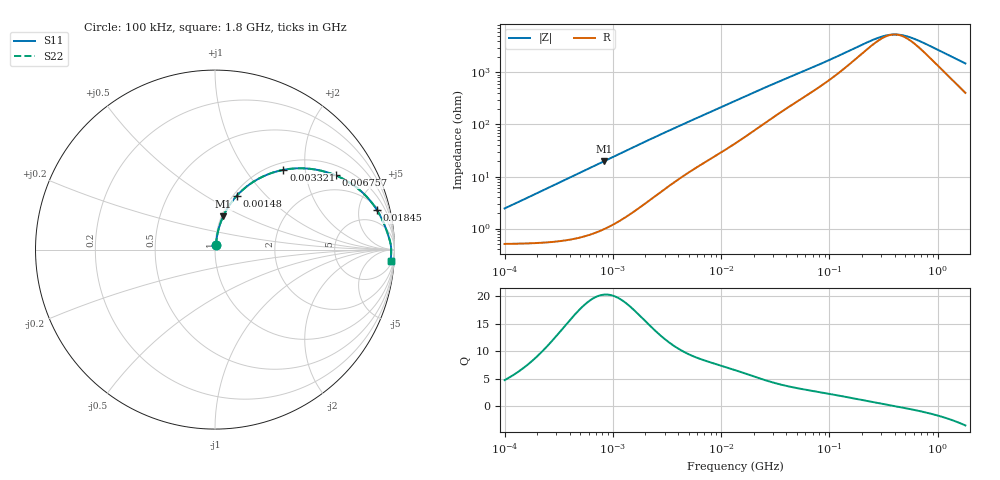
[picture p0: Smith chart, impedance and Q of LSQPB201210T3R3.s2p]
! LSQPB201210T3R3  S-PARAMETER MODEL  ( General Type )
! Model Generated by TAIYO YUDEN Corporation (http://www.ty-top.com)
! Version 2.0
! TAIYO YUDEN Control No. 100810NF18SB-HKC
! Copyright(c) 2007 TAIYO YUDEN CO.,LTD. All Rights Reserved.
! Product Description (link to TY-COMPAS)
! https://ds.yuden.co.jp/TYCOMPAS/or/detail?pn=LSQPB201210T3R3M&u=M
! Products Name : Inductors
! Characteristics :
!  Inductance : 3.3 uH , SRF(min) : 190 MHz , DC Resistance(max) : 0.65 Ohm
!  Rated Current : Saturation :490 mA , Temp Rise : 440 mA (40 degC)
!  Case Size : 2.0 x 1.25 / 0.079 x 0.049 [mm/inch] , Thickness : 1.0 / 0.04 [mm/inch]
!  (Conditions: Temperature = 25 degC , DC Bias Current/Voltage = 0A / 0V)
! External Node Assignments :
!  1  o---GGG---o  2
! GND o---------o GND
! Frequency Range : 0.1MHz  -  1800MHz  [ 402 STEP ]
# MHz S RI R 50
! Freq[MHz].  S11 Real  S11 Imag  S21 Real  S21 Imag  S12 Real  S12 Imag  S22 Real  S22 Imag
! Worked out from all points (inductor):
!   401 points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, 100 kHz to 1.8 GHz, reference 50 ohm
!   read as one part in series: L = 3.8 uH near 105 kHz
!   highest Q = 20.3 at 822 kHz (marker M1), where L = 3.79 uH
!   self-resonance near 395.3 MHz
!   S11 on the Smith chart (normalised r, x): 100 kHz: 1.01, +0.05; 1.48 MHz: 1.04, +0.70; 3.321 MHz: 1.13, +1.53; 6.757 MHz: 1.35, +2.97; 18.45 MHz: 2.34, +7.53; 1.8 GHz: 9, -29
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0.1  0.00561 0.0236  0.9944 -0.0236  0.9944 -0.0236  0.00561 0.0236
0.247521  0.00882 0.0582  0.9912 -0.0582  0.9912 -0.0582  0.00882 0.0582
0.516129  0.0214 0.1196  0.9786 -0.1196  0.9786 -0.1196  0.0214 0.1196
0.822022  0.0454 0.185  0.9546 -0.185  0.9546 -0.185  0.0454 0.185
1.479789  0.1227 0.3014  0.8773 -0.3014  0.8773 -0.3014  0.1227 0.3014
1.985446  0.1948 0.3651  0.8052 -0.3651  0.8052 -0.3651  0.1948 0.3651
2.66389  0.2934 0.4187  0.7066 -0.4187  0.7066 -0.4187  0.2934 0.4187
3.320932  0.3813 0.4443  0.6187 -0.4443  0.6187 -0.4443  0.3813 0.4443
4.679446  0.5275 0.4504  0.4725 -0.4504  0.4725 -0.4504  0.5275 0.4504
6.757206  0.6726 0.4135  0.3274 -0.4135  0.3274 -0.4135  0.6726 0.4135
9.52142  0.7803 0.3525  0.2197 -0.3525  0.2197 -0.3525  0.7803 0.3525
13.41641  0.8561 0.2828  0.1439 -0.2828  0.1439 -0.2828  0.8561 0.2828
18.44729  0.9015 0.2219  0.0985 -0.2219  0.0985 -0.2219  0.9015 0.2219
34.03197  0.9461 0.1329  0.0539 -0.1329  0.0539 -0.1329  0.9461 0.1329
69.24595  0.968 0.0712  0.032 -0.0712  0.032 -0.0712  0.968 0.0712
247.5026  0.9809 0.0138  0.0191 -0.0138  0.0191 -0.0138  0.9809 0.0138
301.0823  0.9813 0.00785  0.0187 -0.00785  0.0187 -0.00785  0.9813 0.00785
357.3983  0.9816 0.00288  0.0184 -0.00288  0.0184 -0.00288  0.9816 0.00288
445.5497  0.9818 -0.00344  0.0182 0.00344  0.0182 0.00344  0.9818 -0.00344
583.3325  0.9818 -0.0114  0.0182 0.0114  0.0182 0.0114  0.9818 -0.0114
763.7235  0.9816 -0.0203  0.0184 0.0203  0.0184 0.0203  0.9816 -0.0203
1800  0.9782 -0.062  0.0218 0.062  0.0218 0.062  0.9782 -0.062
